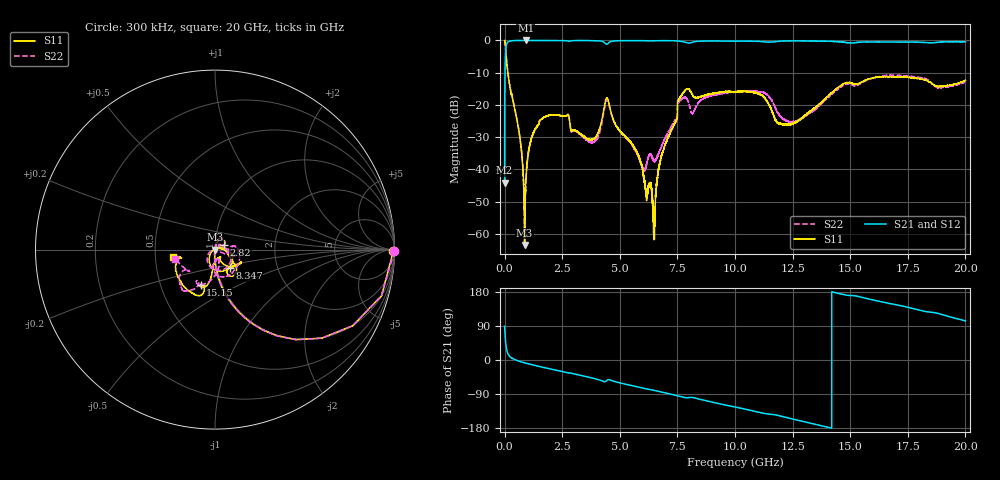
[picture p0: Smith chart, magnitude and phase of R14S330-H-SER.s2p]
!{R14S330}
!Johanson Technology Inc.
!www.johansontechnology.com
!Test Board Conditions:
!Substrate Type  RO4350B
!Substrate Thickness  20 mil
!Substrate Dk  3.66
!TL Type: GCPW
!TL Trace Width  36 mil
!TL Gap  12 mil
!Electrode orientation  Horizontal
!DUT TOPOLOGY	SERIES
!Mounting Pad LxW  26x36 mil
! Created Wed Nov 25 17:33:21 2020
! 2 Port Network Data from SP1.SP block
! freq  magS11  angS11  magS21  angS21  magS12  angS12  magS22  angS22
# khz S ma R 50
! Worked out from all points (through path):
!   20001 points, 300 kHz to 20 GHz, reference 50 ohm
!   highest |S21| = 0.00 dB at 920.3 MHz (marker M1); lowest = -44.1 dB at 300 kHz (marker M2)
!   group delay of S21, straight-line fit = 35.9 ps
!   lowest |S11| = -63.4 dB at 866.3 MHz (marker M3), VSWR 1.00, Z = 50.1 - j0.0381 ohm
!   |S11| at or under -10 dB: 140.4 MHz to end of sweep
!   |S22| runs from -63.8 to 0.0 dB; largest |S21 - S12| = 0.018
!   S11 on the Smith chart (normalised r, x): 300 kHz: open; 2.82 GHz: 1.11, +0.06; 8.347 GHz: 1.15, -0.24; 15.15 GHz: 0.79, -0.32; 20 GHz: 0.62, -0.06
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300  0.9933 -0.6  0.006219 88.9  0.006281 89.2  0.9982 -0.6
128300  0.3442 -71.0  0.9378 19.0  0.9377 18.9  0.3456 -71.0
640300  0.03555 -91.9  0.9985 -3.5  0.9986 -3.5  0.0357 -94.4
866300  0.0006785 -34.1  0.9995 -7.6  0.9998 -7.6  0.001202 -144.3
920300  0.006268 71.4  1 -8.4  0.9994 -8.5  0.006225 91.3
1121300  0.02667 75.2  0.999 -11.6  0.9992 -11.6  0.02604 81.9
1571300  0.05918 71.0  0.9977 -18.1  0.9968 -18.0  0.05916 72.4
2820300  0.0574 27.0  0.9711 -34.2  0.9718 -34.2  0.05521 29.7
3334300  0.03462 38.7  0.9964 -41.0  0.9968 -41.0  0.03362 51.2
3968300  0.03224 18.3  0.9919 -50.2  0.9924 -50.2  0.02854 38.1
4452300  0.1286 -66.2  0.8778 -53.4  0.877 -53.4  0.1203 -71.1
6006300  0.009103 -159.6  0.9922 -74.2  0.9929 -74.2  0.01005 -120.6
6463300  0.001744 -171.5  0.9905 -79.7  0.9901 -79.8  0.0139 -74.7
6667300  0.009264 31.4  0.9925 -82.6  0.9924 -82.6  0.0172 -40.8
7600300  0.1286 -35.2  0.9729 -96.0  0.9729 -95.9  0.1162 8.6
8347300  0.1305 -51.5  0.9671 -101.6  0.9678 -101.5  0.1 10.7
1.00003e7  0.1604 -25.2  0.9748 -123.9  0.975 -123.9  0.1583 -49.4
1.20173e7  0.05121 -54.5  0.9776 -148.6  0.9781 -148.6  0.06463 -87.8
1.33343e7  0.08286 -95.1  0.9786 -167.5  0.9807 -167.6  0.07832 -74.0
1.51513e7  0.212 -112.4  0.9141 169.8  0.9174 169.5  0.1995 -120.1
1.66673e7  0.2728 -115.6  0.9492 149.7  0.9405 149.6  0.2908 -127.2
2e7  0.2402 -169.9  0.9513 103.2  0.9515 103.3  0.2279 -166.7
